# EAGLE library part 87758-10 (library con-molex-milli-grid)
HEADER
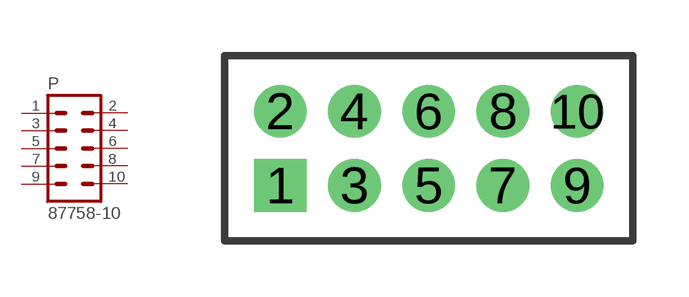
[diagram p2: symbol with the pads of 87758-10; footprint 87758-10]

Designator prefix P

## 87758-10  [87758-10]
1  1  pas
2  2  pas
3  3  pas
4  4  pas
5  5  pas
6  6  pas
7  7  pas
8  8  pas
9  9  pas
10  10  pas

## Footprint 87758-10 (pad centres in mm)
HEADER Dual Row, Vertical
drill 0.914 square: 1 -4,-1
drill 0.914: 2 -4,1; 3 -2,-1; 4 -2,1; 5 0,-1; 6 0,1; 7 2,-1; 8 2,1; 9 4,-1; 10 4,1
